PROGRAM p09_timers
VAR
	pulseTimer: TP;
	onDelayTimer: TON;
	offDelayTimer: TOF;
	ptValue: TIME;
	ontValue: TIME;
	oftValue: TIME;
	S0: BOOL;	
	L0: BOOL;
	L1: BOOL;
	L2: BOOL;
END_VAR

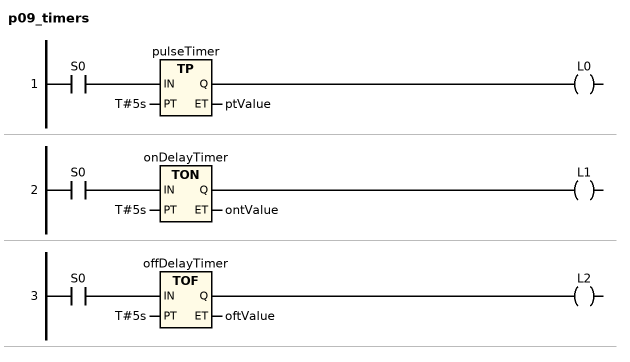
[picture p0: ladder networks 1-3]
// NETWORK 1
pulseTimer(IN := S0, PT := T#5s, ET => ptValue); // TP
L0 := pulseTimer.Q;

// NETWORK 2
onDelayTimer(IN := S0, PT := T#5s, ET => ontValue); // TON
L1 := onDelayTimer.Q;

// NETWORK 3
offDelayTimer(IN := S0, PT := T#5s, ET => oftValue); // TOF
L2 := offDelayTimer.Q;

END_PROGRAM
